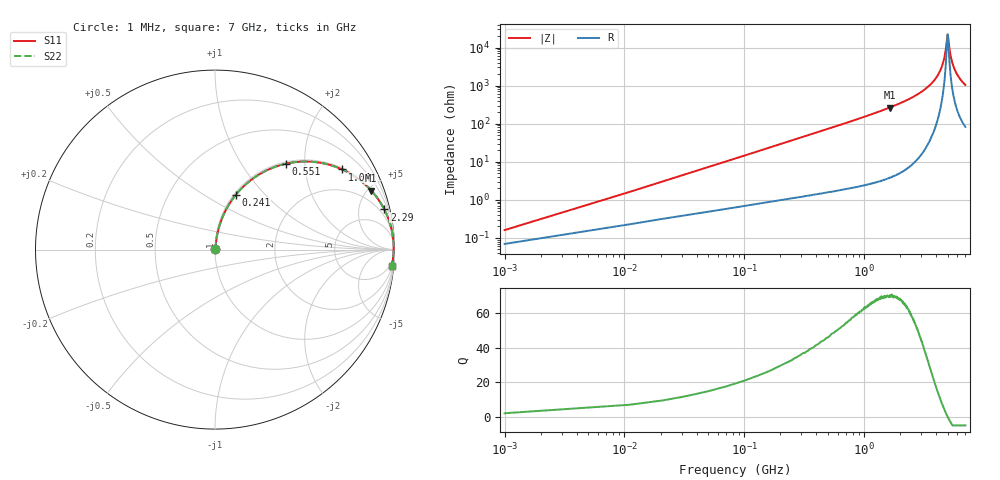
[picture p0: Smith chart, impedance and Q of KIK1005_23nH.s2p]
!version-3
!date-01.2023
!Series
# MHz S RI R 50
!Freq ReS11 ImS11 ReS21 ImS21 ReS12 ImS12 ReS22 ImS22
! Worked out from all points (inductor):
!   701 points, 1 MHz to 7 GHz, reference 50 ohm
!   read as one part in series: L = 23 nH near 31 MHz
!   highest Q = 70 at 1.63 GHz (marker M1), where L = 25.8 nH
!   self-resonance near 4.98 GHz
!   S11 on the Smith chart (normalised r, x): 1 MHz: 1.00, +0.00; 241 MHz: 1.02, +0.70; 551 MHz: 1.03, +1.61; 1.04 GHz: 1.05, +3.15; 2.29 GHz: 1.13, +8.40; 7 GHz: 3, -21
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1  0.000691 0.00144  0.9993 -0.00144  0.9993 -0.00144  0.000691 0.00144
41  0.00785 0.0585  0.9922 -0.0585  0.9922 -0.0585  0.00785 0.0585
61  0.0129 0.0866  0.9871 -0.0866  0.9871 -0.0866  0.0129 0.0866
131  0.0417 0.1801  0.9583 -0.1801  0.9583 -0.1801  0.0417 0.1801
241  0.1161 0.3053  0.8839 -0.3053  0.8839 -0.3053  0.1161 0.3053
371  0.2309 0.4091  0.7691 -0.4091  0.7691 -0.4091  0.2309 0.4091
551  0.3961 0.4789  0.6039 -0.4789  0.6039 -0.4789  0.3961 0.4789
1040  0.7093 0.4463  0.2907 -0.4463  0.2907 -0.4463  0.7093 0.4463
1170  0.7591 0.4202  0.2409 -0.4202  0.2409 -0.4202  0.7591 0.4202
1630  0.871 0.3281  0.129 -0.3281  0.129 -0.3281  0.871 0.3281
2290  0.9432 0.2238  0.0568 -0.2238  0.0568 -0.2238  0.9432 0.2238
2340  0.9465 0.2172  0.0535 -0.2172  0.0535 -0.2172  0.9465 0.2172
3510  0.987 0.0976  0.013 -0.0976  0.013 -0.0976  0.987 0.0976
4230  0.9942 0.0452  0.00584 -0.0452  0.00584 -0.0452  0.9942 0.0452
4670  0.9955 0.0178  0.0045 -0.0178  0.0045 -0.0178  0.9955 0.0178
4800  0.9956 0.0103  0.00442 -0.0103  0.00442 -0.0103  0.9956 0.0103
4940  0.9955 0.00235  0.00448 -0.00235  0.00448 -0.00235  0.9955 0.00235
4990  0.9955 -0.000415  0.00453 0.000415  0.00453 0.000415  0.9955 -0.000415
5180  0.9951 -0.0107  0.00487 0.0107  0.00487 0.0107  0.9951 -0.0107
5330  0.9947 -0.0185  0.00529 0.0185  0.00529 0.0185  0.9947 -0.0185
5840  0.9924 -0.0437  0.00758 0.0437  0.00758 0.0437  0.9924 -0.0437
7000  0.9835 -0.0938  0.0165 0.0938  0.0165 0.0938  0.9835 -0.0938
